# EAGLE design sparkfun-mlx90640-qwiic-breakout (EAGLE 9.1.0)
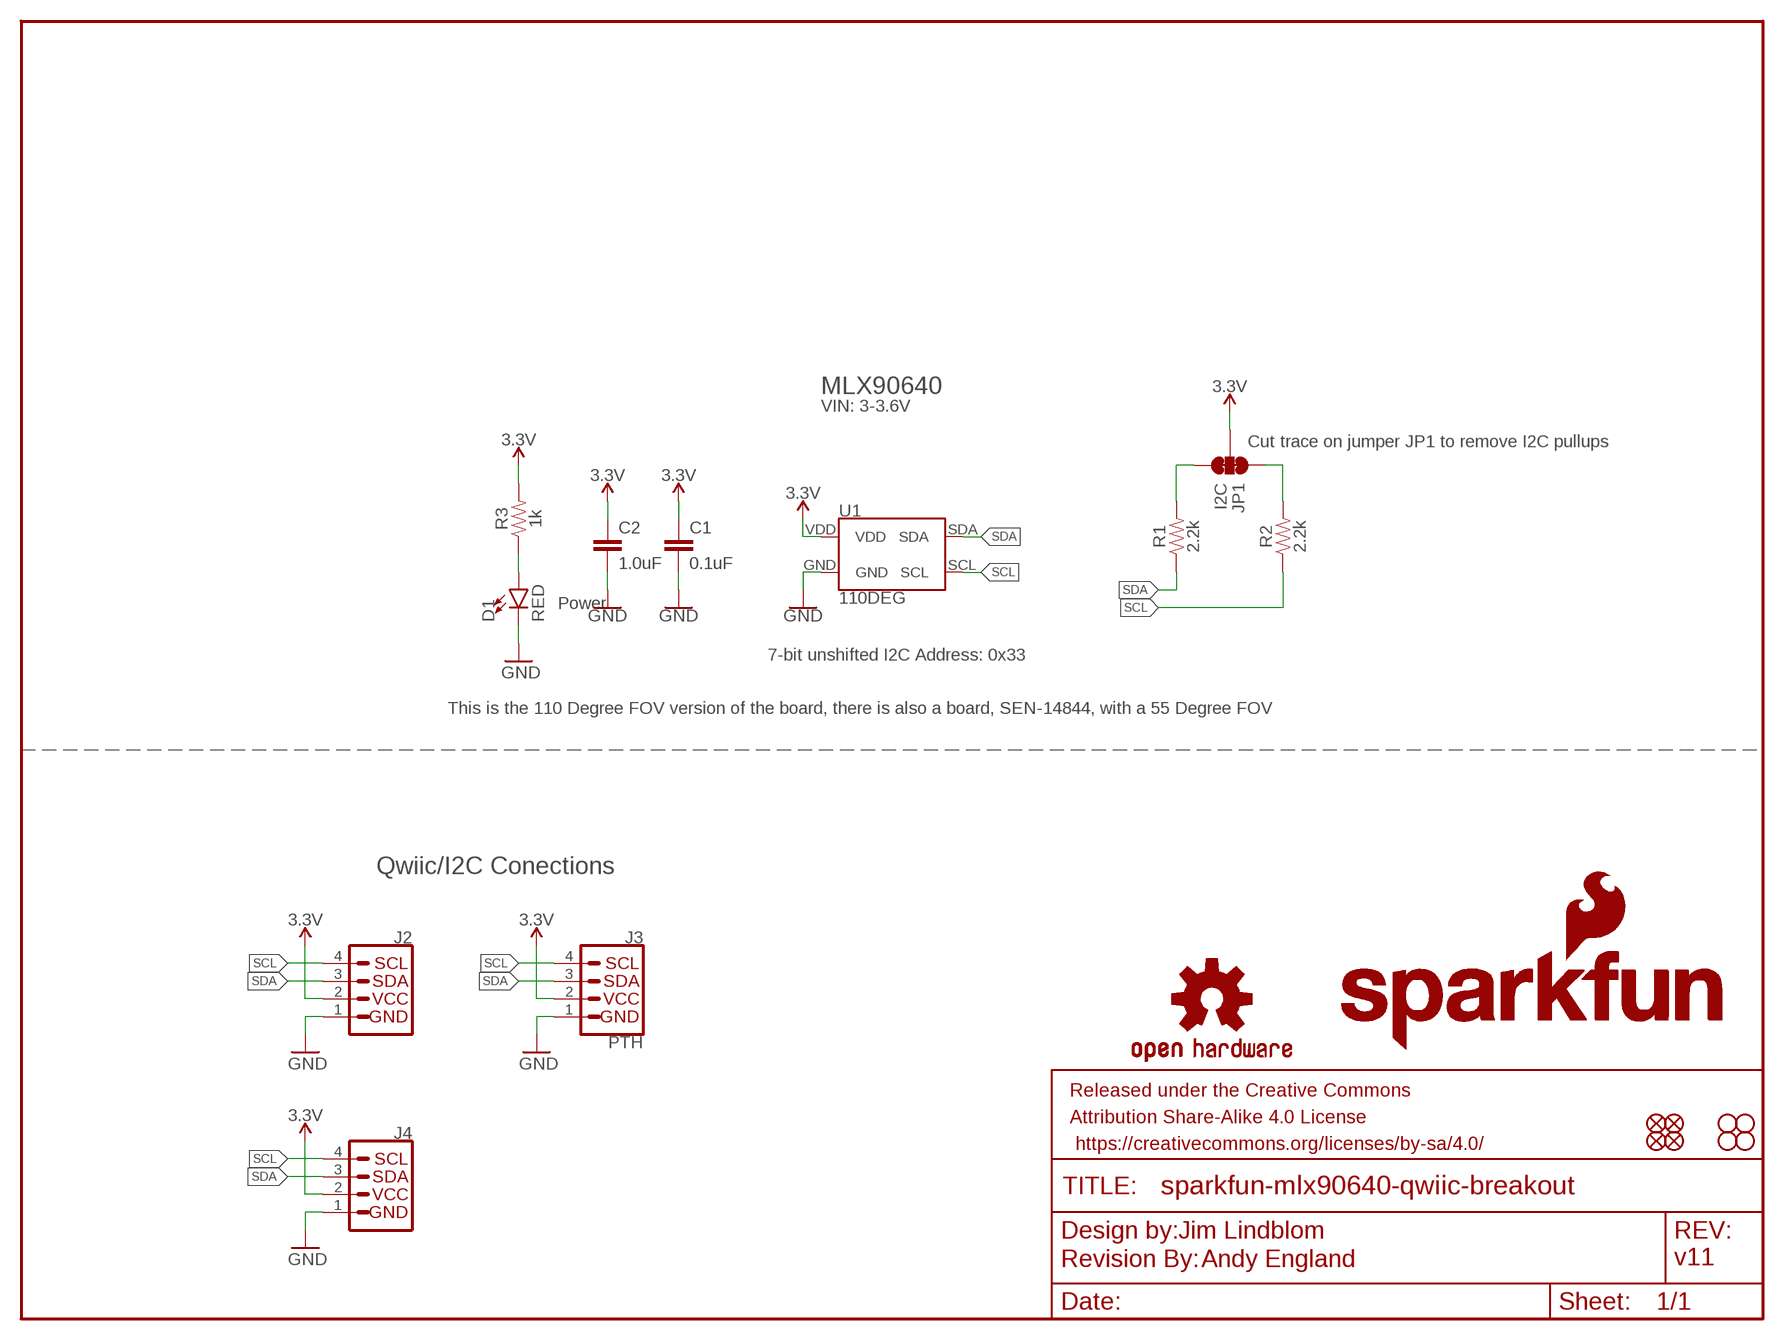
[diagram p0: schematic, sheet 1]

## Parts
C1  0.1uF  0.1UF-0603-25V-(+80/-20%)  [0603]
C2  1.0uF  1.0UF-0603-16V-10%  [0603]
D1  RED  LED-RED0603  [LED-0603]
FRAME1  FRAME-LETTER  [CREATIVE_COMMONS]
J2  QWIIC_CONNECTORJS-1MM  [1X04_1MM_RA]
J3  PTH  I2C_STANDARD_NO_SILK  [1X04_NO_SILK]
J4  QWIIC_CONNECTORJS-1MM  [1X04_1MM_RA]
JP1  I2C  JUMPER-SMT_3_2-NC_TRACE_NO-SILK  [SMT-JUMPER_3_2-NC_TRACE_NO-SILK]
JP2  FIDUCIALUFIDUCIAL  [MICRO-FIDUCIAL]
JP3  STAND-OFF  [STAND-OFF]
JP4  STAND-OFF  [STAND-OFF]
JP5  FIDUCIALUFIDUCIAL  [MICRO-FIDUCIAL]
JP6  FIDUCIALUFIDUCIAL  [MICRO-FIDUCIAL]
JP7  FIDUCIALUFIDUCIAL  [MICRO-FIDUCIAL]
JP8  STAND-OFF  [STAND-OFF]
JP9  STAND-OFF  [STAND-OFF]
LOGO1  OSHW-LOGOMINI  [OSHW-LOGO-MINI]
LOGO2  SFE_LOGO_NAME_FLAME.1_INCH  [SFE_LOGO_NAME_FLAME_.1]
LOGO3  SFE_LOGO_NAME.1_INCH  [SFE_LOGO_NAME_.1]
LOGO4  REVISION  [REVISION]
R1  2.2k  2.2KOHM-0603-1/10W-1%  [0603]
R2  2.2k  2.2KOHM-0603-1/10W-1%  [0603]
R3  1k  1KOHM-0603-1/10W-1%  [0603]
U1  110DEG  MLX90540_MLX906404  [MLX90540_MLX90640]

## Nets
3.3V: C1.1 C2.1 J2.2 J3.2(VCC) J4.2 JP1.2 R3.2 U1.VDD
GND: C1.2 C2.2 D1.C J2.1 J3.1(GND) J4.1 U1.GND
N$1: JP1.3 R1.2
N$2: JP1.1 R2.2
N$3: D1.A R3.1
SCL: J2.4 J3.4(SCL) J4.4 R2.1 U1.SCL
SDA: J2.3 J3.3(SDA) J4.3 R1.1 U1.SDA

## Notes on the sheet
- MLX90640
- VIN: 3-3.6V
- Cut trace on jumper JP1 to remove I2C pullups
- Power
- 7-bit unshifted I2C Address: 0x33
- This is the 110 Degree FOV version of the board, there is also a board, SEN-14844, with a 55 Degree FOV
- Qwiic/I2C Conections
- Jim Lindblom
- Andy England | v11

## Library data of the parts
C1 = SparkFun-Capacitors:0.1UF: 0.1µF ceramic capacitors; PROD_ID: CAP-00810
C2 = SparkFun-Capacitors:1.0UF: 1µF ceramic capacitors; PROD_ID: CAP-00868
D1 = SparkFun-LED:LED-RED: Red SMD LED; PROD_ID: DIO-00819
FRAME1 = SparkFun-Aesthetics:FRAME-LETTER: Schematic Frame - Letter
J2 J4 = SparkFun-Connectors:QWIIC_CONNECTOR: SparkFun I2C Standard Qwiic Connector An SMD 1mm pitch JST connector makes it easy and quick (get it? Qwiic?) to connect I2C devices to each other. The Qwiic system enables fast and solderless connection between popular platforms and various sensors and actuators. We carry 200mm, 100mm, 50mm, and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; PROD_ID: CONN-13694
J3 = SparkX:I2C_STANDARD: SparkFun I2C Standard Pinout Header SparkFun has standardized on a pinout for all I2C based sensor breakouts. This pinout allows I2C boards to be plugged directly into the headers on Arduino Uno compatible boards, and to be daisy chained easily. Example SparkFun Products: SparkFun Atmospheric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
JP1 = SparkFun-Jumpers:JUMPER-SMT_3_2-NC_TRACE: Normally closed trace jumper (2 of 2 connections) This jumper has a trace between all three pads so they are normally closed (NC). Use a razor knife to open the connection(s). For best results follow the IPC guidelines for cutting traces: Cutout at least 0.063 mm (0.005 in). Remove all loose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
JP2 JP5-JP7 = SparkFun:FIDUCIAL: Fiducial Alignment Points
JP3 JP4 JP8 JP9 = SparkFun:STAND-OFF: Stand Off
LOGO1 = SparkFun-Aesthetics:OSHW-LOGO: Open-Source Hardware (OSHW) Logo
LOGO2 = SparkFun-Aesthetics:SFE_LOGO_NAME_FLAME: SparkFun Font Logo w/ Flame
LOGO3 = SparkFun-Aesthetics:SFE_LOGO_NAME: SparkFun Font Logo
LOGO4 = SparkFun-Aesthetics:REVISION: "Revision By" Text
R1 R2 = SparkFun-Resistors:2.2KOHM: 2.2kΩ resistor; PROD_ID: RES-08272
R3 = SparkFun-Resistors:1KOHM: 1kΩ resistor; PROD_ID: RES-07856
U1 = SparkFun-IC-Special-Function:MLX90540_MLX90640: Melexis MLX90640 Infrared Array The MLX90640 is a fully calibrated 32x24 pixels thermal IR array in an industry standard 4-lead TO39 package with digital interface.; PROD_ID: IC-14041

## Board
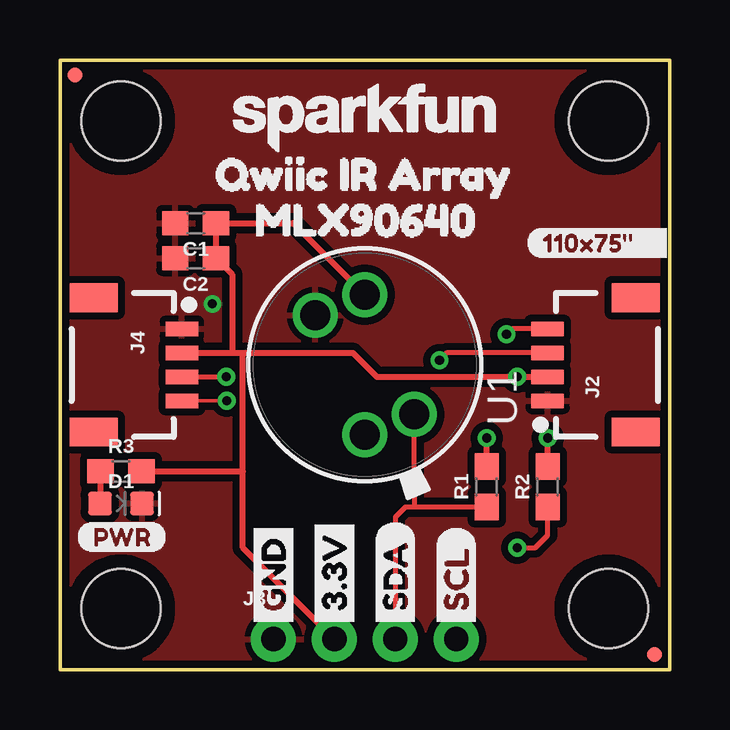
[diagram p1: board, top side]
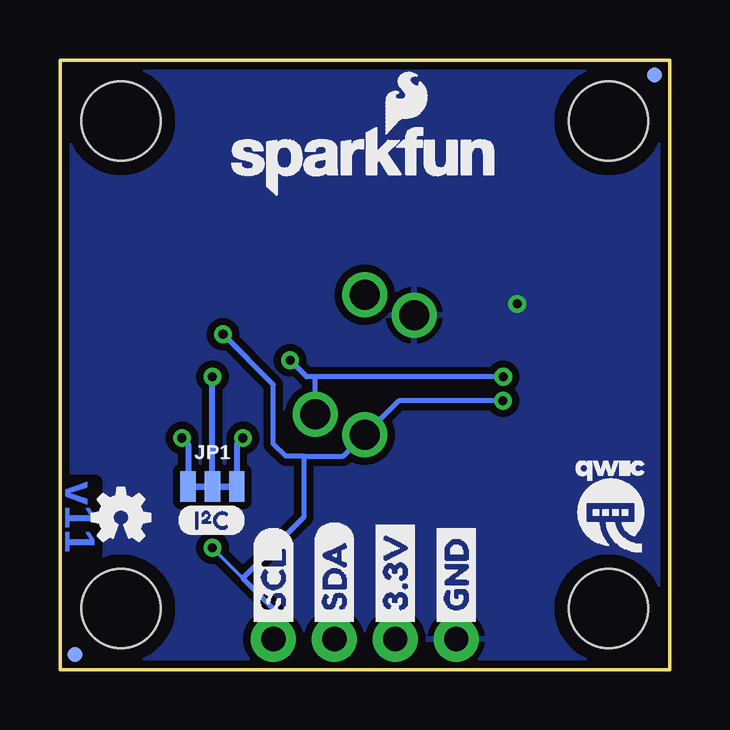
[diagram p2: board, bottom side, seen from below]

Size 25.4 x 25.4 mm. Coordinates in mm from the lower left corner, seen from the top.
Outline: 0,0 25.4,0 25.4,25.4 0,25.4 0,0
Copper layers (1*16): Top 0.035mm / dielectric 1.5mm / Bottom 0.035mm
Design rules "SparkFun-2-layer-TIGHT": minimum track width 7mil, minimum drill 15mil, track to track 7mil, track to pad 7mil, pad to pad 7mil, via to via 7mil, smd to smd 7mil, copper to edge 7mil, drill to drill 7mil, minimum pad ring 7mil, minimum via ring 7mil, stop-mask expansion 4mil, vias tented up to drill 25mil, thermal gap 10mil

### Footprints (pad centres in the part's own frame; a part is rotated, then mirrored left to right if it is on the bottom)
0603 = smd 1.1 x 1: 1 -0.85,0; 2 0.85,0
LED-0603 = smd 1 x 1: A -0.877,0; C 0.877,0
1X04_1MM_RA = smd 0.6 x 1.35: 1 -1.5,0; 2 -0.5,0; 3 0.5,0; 4 1.5,0 | smd 1.2 x 2: NC1 2.8,-3.675; NC2 -2.8,-3.675
1X04_NO_SILK = drill 1.016 pad 1.88: 1 0,0; 2 2.54,0; 3 5.08,0; 4 7.62,0
SMT-JUMPER_3_2-NC_TRACE_NO-SILK = smd 0.635 x 1.27: 1 -1.016,0; 2 0,0; 3 1.016,0
MICRO-FIDUCIAL = smd 0.635 x 0.635: 1 0,0
STAND-OFF = hole 3.302: 0,0
MLX90540_MLX90640 = drill 1.25: GND 2.065,2.065; SCL -2.92,0; SDA -2.065,-2.065; VDD 2.92,0

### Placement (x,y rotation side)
C1  5.65,18.61 180 top
C2  5.65,17.14 180 top
D1  2.54,6.92 0 top
FRAME1  not placed on the board
J2  20.32,12.7 90 top
J3  8.89,1.27 0 top
J4  5.08,12.7 270 top
JP1  19.05,7.62 0 bottom
JP2  24.77,0.64 0 top
JP3  2.54,22.86 0 top
JP4  22.86,22.86 0 top
JP5  0.64,24.77 0 top
JP6  24.77,0.64 0 bottom
JP7  0.64,24.77 0 bottom
JP8  2.54,2.54 0 top
JP9  22.86,2.54 0 top
LOGO1  22.86,6.35 0 bottom
LOGO2  18.67,19.68 0 bottom
LOGO3  6.73,21.08 0 top
LOGO4  not placed on the board
R1  17.78,7.62 90 top
R2  20.32,7.62 90 top
R3  2.54,8.26 0 top
U1  12.7,12.7 90 top
U$1  [SDA-[)]  13.97,1.52 90 top
U$2  [110X75#____0]  19.43,17.78 0 top
U$4  [SCL-[)]  16.51,1.52 90 top
U$5  [3.3V]  11.43,1.52 90 top
U$6  [GND-04]  8.89,1.52 90 top
U$7  [SDA-[)]  13.97,1.52 90 bottom
U$8  [SCL-[)]  16.51,1.52 90 bottom
U$9  [3.3V]  11.43,1.52 90 bottom
U$10  [GND-04]  8.89,1.52 90 bottom
U$11  [QWIIC-LOGO-SMALL]  2.54,6.79 0 bottom
U$12  [PWR-()-03]  0.7,5.52 0 top
U$13  [MLX906401]  6.99,18.73 0 top
U$14  [QWIIC_IR_ARRAY0]  5.33,20.64 0 top
U$16  [I_SUPER2_C-()-03]  20.51,6.22 0 bottom

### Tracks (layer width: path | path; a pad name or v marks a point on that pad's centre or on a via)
3.3V  (via drill 0.38)
  Top 0.254: J4.2 7.18,13.2 | 7.18,13.2 7.62,13.2 | 7.62,13.2 12.2,13.2 13.2,12.2 v19.05,12.2 J2.2 | J3.2 7.62,5.08 7.62,8.26 | 7.62,8.26 7.62,13.2 | R3.2 7.62,8.26 | 7.18,13.2 7.18,16.47 C2.1 C1.1 9.71,18.61 U1.VDD
  Bottom 0.254: JP1.2 v19.05,12.2
GND  (via drill 0.38)
  other vias: 6.35,15.24
  pour Top (isolate 0.305): 0,0 0,25.4 25.4,25.4 25.4,0
  pour Bottom (isolate 0.305): 0,0 0,25.4 25.4,25.4 25.4,0
N$1  (via drill 0.38)
  Top 0.254: R1.2 v17.78,9.65
  Bottom 0.254: v17.78,9.65 18.03,9.4 JP1.3
N$2  (via drill 0.38)
  Top 0.254: R2.2 v20.32,9.65
  Bottom 0.254: v20.32,9.65 20.07,9.4 JP1.1
N$3
  Top 0.254: D1.A 1.69,6.95 R3.1
SCL  (via drill 0.38)
  Top 0.152: J4.4 v6.95,11.2
  Top 0.203: J2.4 18.84,14.2 v18.61,13.97 | v19.05,5.08 19.81,5.08 20.32,5.59 R2.1
  Bottom 0.152: 17.78,3.81 v19.05,5.08
  Bottom 0.203: v6.95,11.2 11.28,11.2 U1.SCL 13.59,8.89 15.24,8.89 | v18.61,13.97 16.51,11.87 16.51,9.4 16,8.89 15.24,8.89 | J3.4 16.51,2.54 17.78,3.81 15.24,6.35 15.24,8.89
SDA  (via drill 0.38)
  Top 0.152: 14.77,6.78 14.76,6.77
  Top 0.203: J4.3 v6.93,12.2 | J2.3 16.12,13.2 v15.81,12.89 | R1.1 15.99,6.77 14.76,6.77 14.39,6.77 13.97,6.35 J3.3 | U1.SDA 14.77,7.38 14.77,6.78
  Bottom 0.203: v6.93,12.2 14.77,12.2 | 14.77,12.2 15.12,12.2 v15.81,12.89 | U1.SDA 14.77,12.2

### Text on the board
Bottom: v11
Measures: Units in In.
tDocu: Jim Lindblom | Andy England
